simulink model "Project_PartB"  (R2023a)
settings: Solver=FixedStepAuto  StartTime=0.0  StopTime=inf  FixedStep=.01  RelTol=1e-3  EnableMultiTasking=on
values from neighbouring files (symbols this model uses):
  encoderResolution = 48    [project_constants.m]
  gearRatio = 171.79    [project_constants.m]
libraries: arduinolib x4, arduinosensorlib x1

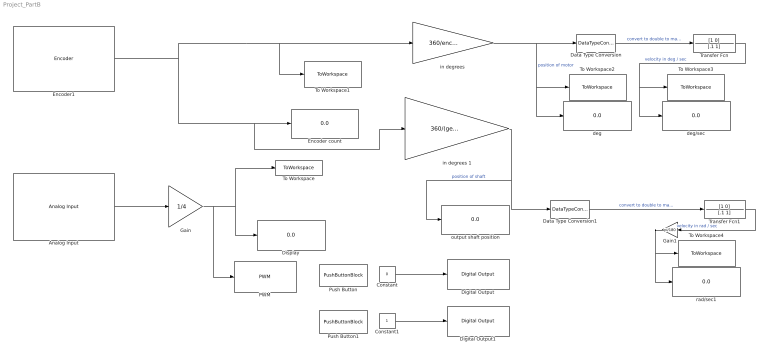
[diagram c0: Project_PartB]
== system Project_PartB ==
  Analog Input : arduinolib/Analog Input  pinNumber=0  ReadResultsOnly=off  ConversionTriggerSource=Software  ExternalTriggerType=uint32( 0 )  OutputDataType=uint16  EnableConversionCompleteNotify=off  EnableOuputStatus=off  SampleTime=-1  blockPlatform=arduino
  Constant : Constant  Value=0
  Constant1 : Constant
  Data Type Conversion : DataTypeConversion  OutDataTypeStr=double
  Data Type Conversion1 : DataTypeConversion  OutDataTypeStr=double
  Digital Output : arduinolib/Digital Output  pinNumber=10  Direction=output  blockPlatform=arduino
  Digital Output1 : arduinolib/Digital Output  pinNumber=11  Direction=output  blockPlatform=arduino
  Display : Display
  Encoder count : Display
  Encoder1 : arduinosensorlib/Encoder  InputA=2  InputB=3  Mode=No reset  SampleTime=-1
  Gain : Gain  Gain=1/4
  Gain1 : Gain  Gain=pi/180
  PWM : arduinolib/PWM  pinNumber=9  frequencyType=Default  desiredFrequency=490.2  achievableFrequency=490.2
  Push Button : PushButtonBlock  ButtonText=Pin2  OnValue=0  ButtonType=Latch  OffValue=1.000000
  Push Button1 : PushButtonBlock  ButtonText=Pin7  OnValue=0  ButtonType=Latch  OffValue=1.000000
  To Workspace : ToWorkspace  VariableName=pot_reading  SaveFormat=Structure With Time  SampleTime=-1
  To Workspace1 : ToWorkspace  VariableName=encoder_reading  SaveFormat=Structure With Time  SampleTime=-1
  To Workspace2 : ToWorkspace  VariableName=position  SaveFormat=Structure With Time  SampleTime=-1
  To Workspace3 : ToWorkspace  VariableName=speed  SaveFormat=Structure With Time  SampleTime=-1
  To Workspace4 : ToWorkspace  VariableName=shaft_speed  SaveFormat=Structure With Time  SampleTime=-1
  Transfer Fcn : TransferFcn  Numerator=[1 0]  Denominator=[.1 1]
  Transfer Fcn1 : TransferFcn  Numerator=[1 0]  Denominator=[.1 1]
  deg : Display
  deg/sec : Display
  "in degrees " : Gain  Gain=360/encoderResolution
  in degrees 1 : Gain  Gain=360/(gearRatio*encoderResolution)
  output shaft position : Display
  rad/sec1 : Display
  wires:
  Analog Input/1 -> Gain/1
  Gain/1 -> PWM/1, To Workspace/1, Display/1
  Encoder1/1 -> "in degrees "/1, To Workspace1/1, in degrees 1/1, Encoder count/1
  Transfer Fcn/1 -> deg/sec/1, To Workspace3/1  "velocity in deg / sec"
  Data Type Conversion/1 -> Transfer Fcn/1  "convert to double to make TF happy"
  "in degrees "/1 -> Data Type Conversion/1, deg/1, To Workspace2/1  "position of motor"
  in degrees 1/1 -> Data Type Conversion1/1, output shaft position/1  "position of shaft"
  Constant/1 -> Digital Output/1
  Constant1/1 -> Digital Output1/1
  Transfer Fcn1/1 -> Gain1/1  "velocity in rad / sec"
  Data Type Conversion1/1 -> Transfer Fcn1/1  "convert to double to make TF happy"
  Gain1/1 -> rad/sec1/1, To Workspace4/1
